ORGANIZATION_BLOCK MAIN:OB1
TITLE= Ciclo Automatico per due unità operatrici
// Simulatore: 03
// Versione: 1.0
// Data: 28/02/2002
//
//------------- Descrizione del controllo ---------------
// Il programma svolge il controllo di un ciclo automatico
// la cui sequenza operativa prevede:
// 1) Ciclo 1 - la prima unità operatrice (motore M1) deve
// essere avviata a tensione ridotta (Stella/Triangolo)
// mediante il pulsante SB2 e in seguito arrestata
// manualmente mediante il pulsante SB1.
// 2) Ciclo 2 - dopo quattro arresti manuali della prima
// unità deve intervenire automaticamente la seconda
// unità (motore M2) per un tempo prefissato (10 s)
// trascorso il quale l'unità si arresta automaticamente.
// 3) Durante il ciclo 2 deve essere impedita l'inserzione
// della prima unità operatrice.
// 4) L'inserzione della seconda unità può essere eseguita
// manualmente tramite il pulsante SB3.
// Il tempo di commutazione (Y-D) e quello di lavoro della
// seconda unità sono ottenuti mediante due temporizzatori
// software (T33-T34). Per il conteggio delle inserzioni
// consecutive della prima unità è previsto un contatore
// software C0.
// Nel sistema è previsto un arresto di emergenza simulato
// dal pulsante SB4 il cui intervento porta all'arresto
// delle due unità.
// Ogni unità verrà anche arrestata automaticamente in caso
// di intervento del rispettivo relè termico.
// Per ogni unità sono previste tre lampade che segnalano
// rispettivamente la marcia del motore, l'arresto e l'intervento
// del relè termico.

BEGIN
NETWORK 1 //Marcia-Arresto Motore M1
//
LD Q0.0
A I0.2
O I0.1
A I0.0
AN I0.4
A I1.0
A I0.5
= Q0.0

NETWORK 2 //Gestione Fase Stella Motore M1
//
LDN T33
A I0.2
AN I0.6
= Q0.1

NETWORK 3 //Temporizzatore Stella
//
LDN Q0.2
A Q0.0
TON T33 +50

NETWORK 4 //Gestione Fase Triangolo Motore M1
//
LD T33
O Q0.2
A I0.2
AN I0.7
= Q0.2

NETWORK 5 //Contatore cicli Motore M1
//
LD Q0.2
ED
LD T34
CTU C0 +3

NETWORK 6 //Marcia Motore M2
//
LD Q0.3
A I0.4
O I0.3
O C0
AN T34
A I1.1
AN I0.2
A I0.5
= Q0.3

NETWORK 7 //Temporizzatore Marcia Motore M2
//
LD Q0.3
TON T34 +100

NETWORK 8 //Segnalazione Arresto Motore M1
//
LDN Q0.0
= Q0.4

NETWORK 9 //Segnalazione Marcia Motore M1
//
LD Q0.0
= Q0.5

NETWORK 10 //Segnalazione intervento Relè Termico Motore M1
//
LDN I1.0
= Q1.0

NETWORK 11 //Segnalazione Arresto Motore M2
//
LDN Q0.3
= Q0.6

NETWORK 12 //Segnalazione Marcia Motore M2
//
LD Q0.3
= Q0.7

NETWORK 13 //Segnalazione intervento Relè Termico Motore M2
//
LDN I1.1
= Q1.1

END_ORGANIZATION_BLOCK

